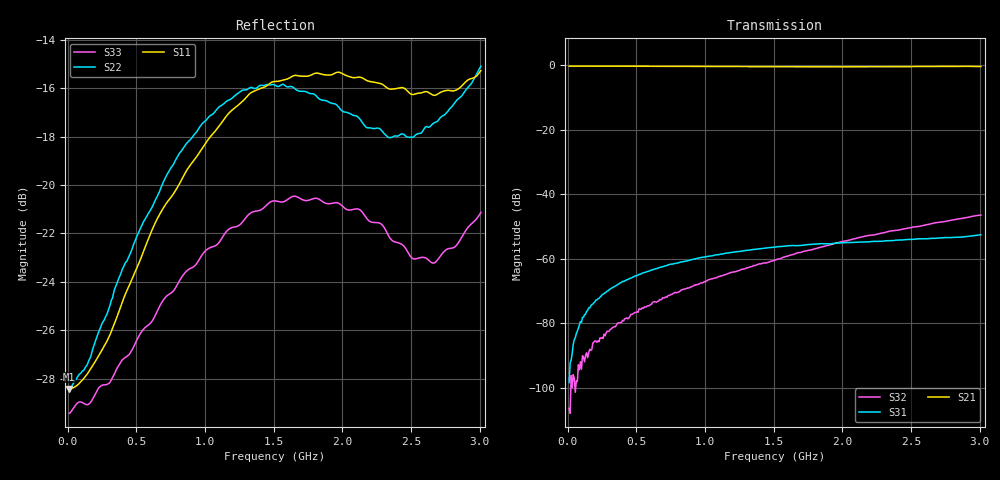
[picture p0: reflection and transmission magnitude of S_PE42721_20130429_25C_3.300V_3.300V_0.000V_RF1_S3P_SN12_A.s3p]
! Device ID: PE42721_20130429
! Serial: 12
! Insertion: A
! Temp: 25C
! VDD: 3.300
! Control_Hi: 3.300
! Control_Lo: 0.000
! Logic State: RF1
! ThroughPath: 2-1
! Port 1: RFC
! Port 2: RF1
! Port 3: RF2
! V1 = 3.30
! V2 = 3.30
! V3 = 0.00
! IDD: 1.054739e-04
! FILE NAME
! DATE 04-30-2013 12:02:46
! CORRECTED  DATA
#  Hz  S  RI  R  75
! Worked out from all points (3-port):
!   401 points, 10 MHz to 3.01 GHz, reference 75 ohm
!   strongest paths, dB at 10 MHz, 760 MHz, 1.51 GHz, 2.26 GHz, 3.01 GHz:
!     S21: -0.4, -0.4, -0.5, -0.6, -0.5
!     S31: -98.3, -61.7, -56.3, -54.6, -52.6
!     S32: -106.3, -71.0, -60.4, -52.3, -46.5
!   lowest |S11| = -28.4 dB at 10 MHz (marker M1), VSWR 1.08, Z = 80.9 - j0.224 ohm
!   |S11| at or under -10 dB: start of sweep to end of sweep
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1e7  0.0379 -0.00138  0.9559 -0.00217  -4.42e-06 1.29e-05
     0.9564 -0.00203  0.0379 -0.00145  1.86e-07 -5.95e-06
     7.9e-06 9.19e-06  -1.99e-08 -4.84e-06  0.0338 -0.000558
8.5e7  0.0374 -0.011  0.9558 -0.0173  -1.68e-06 9.48e-05
       0.9562 -0.0171  0.0391 -0.0112  -4.66e-06 -2.02e-05
       -1.48e-06 9.53e-05  -8.81e-06 -1.7e-05  0.0354 -0.00455
1.9e8  0.0355 -0.0239  0.9549 -0.0387  -1.64e-06 0.000208
       0.9555 -0.0385  0.0389 -0.0256  -2.42e-05 -3.58e-05
       -1.14e-06 0.000208  -2.44e-05 -4.54e-05  0.0348 -0.0112
3.7e8  0.0281 -0.0467  0.9514 -0.0753  -1.96e-05 0.000405
       0.9525 -0.0751  0.0393 -0.0506  -7.12e-05 -7.55e-05
       -1.97e-05 0.000405  -7.11e-05 -7.31e-05  0.0362 -0.022
5.275e8  0.0209 -0.0668  0.9471 -0.1071  -4.49e-05 0.00058
         0.9478 -0.1068  0.0394 -0.071  -0.000134 -8.93e-05
         -3.9e-05 0.000572  -0.000134 -9.95e-05  0.038 -0.0314
9.85e8  -0.00708 -0.1195  0.9263 -0.1925  -0.000124 0.00105
        0.9269 -0.1941  0.0289 -0.1311  -0.000396 -0.00016
        -0.000123 0.00106  -0.000395 -0.000159  0.0461 -0.0555
1.51e9  -0.0152 -0.1628  0.8953 -0.2852  -0.000265 0.0015
        0.8955 -0.2866  -0.00612 -0.1605  -0.000903 -0.000305
        -0.000268 0.0015  -0.000904 -0.000314  0.0589 -0.0716
2.1175e9  0.00486 -0.1668  0.8515 -0.3872  -0.000538 0.00173
          0.8526 -0.3857  -0.0528 -0.1273  -0.00205 -0.000535
          -0.00054 0.00173  -0.00205 -0.000541  0.0554 -0.0699
2.5e9  0.000342 -0.154  0.8244 -0.4542  -0.000876 0.00179
       0.8275 -0.454  -0.0748 -0.1008  -0.00296 -0.0006
       -0.000886 0.00179  -0.00298 -0.000613  0.0315 -0.0637
3.01e9  -0.0749 -0.155  0.7588 -0.5641  -0.00156 0.00178
        0.7644 -0.5538  -0.1134 -0.1343  -0.00472 -0.00049
        -0.00156 0.00177  -0.00472 -0.000454  -0.0199 -0.0855
